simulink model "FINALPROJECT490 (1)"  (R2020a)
settings: Solver=VariableStepAuto  StartTime=0.0  StopTime=4/60  RelTol=1e-3
libraries: powerlib x11, powerlib_meascontrol x9

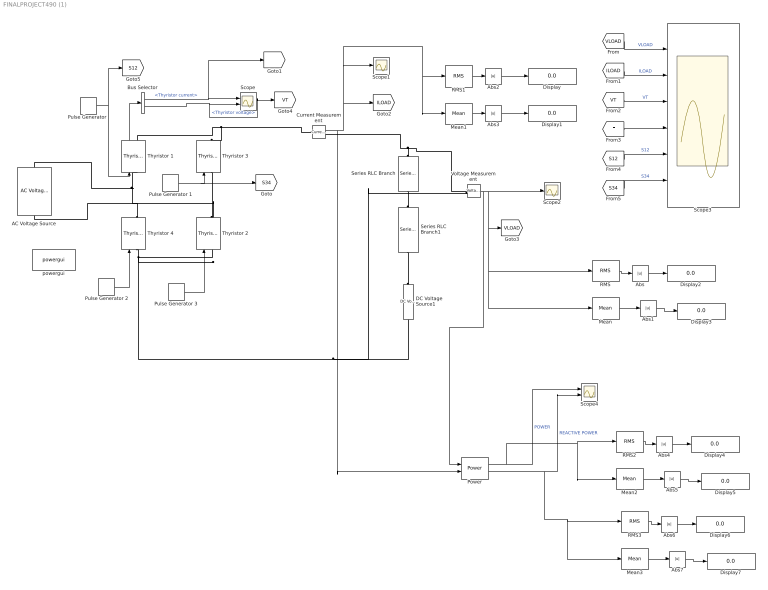
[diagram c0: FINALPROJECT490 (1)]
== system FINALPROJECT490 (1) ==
  "AC Voltage Source " : powerlib/Electrical Sources/AC Voltage Source  Amplitude=169.7  Phase=0  Frequency=60  SampleTime=0  Measurements=None  BusType=swing  Pref=10e3  Qref=0  Qmin=-inf  Qmax=+inf
  Abs{,1..7} (8 alike) : Abs
  Bus Selector : BusSelector  OutputSignals=Thyristor current,Thyristor voltage
  Current Measurement : powerlib/Measurements/Current Measurement  PhasorSimulation=off  OutputType=Complex  PSBequivalent=0
  DC Voltage Source1 : powerlib/Electrical Sources/DC Voltage Source  Amplitude=100  Measurements=None
  Display{,1..7} (8 alike) : Display
  Mean{,1..3} (4 alike) : powerlib_meascontrol/Measurements/Mean  Freq=60  Vinit=0  Ts=0
  Power : powerlib_meascontrol/Measurements/Power  Freq=60  Vinit=[1, 0]  Iinit=[1, 0]  Ts=0
  "Pulse Generator " : DiscretePulseGenerator  PulseType=Time based  Amplitude=5  Period=1/60  PulseWidth=0.51/60  PhaseDelay=((141/360)/60)
  Pulse Generator 1 : DiscretePulseGenerator  PulseType=Time based  Amplitude=5  Period=1/60  PulseWidth=0.51/60  PhaseDelay=(141/360/60)+(0.5/60)
  Pulse Generator 2 : DiscretePulseGenerator  PulseType=Time based  Amplitude=5  Period=1/60  PulseWidth=0.51/60  PhaseDelay=(141/360/60)+(0.5/60)
  Pulse Generator 3 : DiscretePulseGenerator  PulseType=Time based  Amplitude=5  Period=1/60  PulseWidth=0.51/60  PhaseDelay=((141/360)/60)
  RMS{,1..3} (4 alike) : powerlib_meascontrol/Measurements/RMS  TrueRMS=on  Freq=60  RMSInit=120  Ts=0
  Scope : Scope  NumInputPorts=2
  Scope1 : Scope
  Scope2 : Scope
  Scope3 : Scope  NumInputPorts=6
  Scope4 : Scope  NumInputPorts=2
  Series RLC Branch : powerlib/Elements/Series RLC Branch  LConnTagsString=__new0  RConnTagsString=__new0  BranchType=R  Resistance=0.8  Inductance=1e-3  SetiL0=off  InitialCurrent=0  Capacitance=1e-6  Setx0=off  InitialVoltage=0  Measurements=None
  Series RLC Branch1 : powerlib/Elements/Series RLC Branch  LConnTagsString=__new0  RConnTagsString=__new0  BranchType=L  Resistance=20  Inductance=.117  SetiL0=off  InitialCurrent=0  Capacitance=1e-6  Setx0=off  InitialVoltage=0  Measurements=None
  "Thyristor 1 " : powerlib/Power Electronics/Thyristor  Ron=0.001  Lon=0  Vf=0.001  IC=0  Rs=0  Cs=0  Measurements=on
  "Thyristor 2 " : powerlib/Power Electronics/Thyristor  Ron=0.001  Lon=0  Vf=0.001  IC=0  Rs=0  Cs=0  Measurements=on
  "Thyristor 3 " : powerlib/Power Electronics/Thyristor  Ron=0.001  Lon=0  Vf=0.001  IC=0  Rs=0  Cs=0  Measurements=on
  "Thyristor 4 " : powerlib/Power Electronics/Thyristor  Ron=0.001  Lon=0  Vf=0.001  IC=0  Rs=0  Cs=0  Measurements=on
  Voltage Measurement : powerlib/Measurements/Voltage Measurement  PhasorSimulation=off  OutputType=Complex  PSBequivalent=0
  powergui : powerlib/powergui  Priority=1  SimulationMode=Continuous  SampleTime=50e-6  frequency=60  Iterations=50  frequencyindice=60  Pbase=100e6  ErrMax=1e-4  UnitsV=kV  UnitsW=MW  buscounter=0  FunctionMessages=off  echomessages=off  EnableUseOfTLC=off  CurrentSourceSwitches=off  DisableSnubberDevices=off  DisableRonSwitches=off  DisableVfSwitches=off  DisplayEquations=off  AutomaticDiscreteSolvers=off  SolverType=Tustin/Backward Euler (TBE)  Interpol=off  ExternalGateDelay=off  methode=off  Ts=100  x0status=blocks  SPID=on  SwTol=0  HookPort=off  NonlinearTolerance=1e-4  nMaxIteration=100  ContinueOnMaxIteration=off  RestoreLinks=warning  ResistiveCurrentMeasurement=off  Frange=[0:2:500]  Ylog=off  Xlog=on  ShowGrid=off  save=off  variable=ZData  structure=Scope6inputs  ZoomFFT=off  StartTime=0.0  cycles=1  DisplayStyle=4  fundamental=60  FreqAxis=off  MaxFrequency=1000  frequencyindicesteady=1  RmsSteady=1  display=off
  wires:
  Pulse Generator 1/1 -> [S34], "Thyristor 3 "/1
  "Pulse Generator "/1 -> [S12], "Thyristor 1 "/1
  RMS1/1 -> Abs2/1
  Pulse Generator 3/1 -> "Thyristor 2 "/1
  Pulse Generator 2/1 -> "Thyristor 4 "/1
  Abs3/1 -> Display1/1
  Mean1/1 -> Abs3/1
  Bus Selector/1 -> [IT], Scope/1  "<Thyristor current>"
  Abs2/1 -> Display/1
  [ILOAD] -> Scope3/2  "ILOAD"
  RMS/1 -> Abs/1
  [IT] -> Scope3/4  "IT"
  [S34] -> Scope3/6  "S34"
  Bus Selector/2 -> [VT], Scope/2  "<Thyristor voltage>"
  Current Measurement/1 -> Power/2, Scope1/1, Mean1/1, RMS1/1, [ILOAD]
  "Thyristor 1 "/1 -> Bus Selector/1
  [VT] -> Scope3/3  "VT"
  Abs/1 -> Display2/1
  [VLOAD] -> Scope3/1  "VLOAD"
  Voltage Measurement/1 -> Scope2/1, Mean/1, RMS/1, [VLOAD], Power/1
  [S12] -> Scope3/5  "S12"
  Mean/1 -> Abs1/1
  Abs1/1 -> Display3/1
  Abs4/1 -> Display4/1
  RMS2/1 -> Abs4/1
  Abs5/1 -> Display5/1
  Mean2/1 -> Abs5/1
  RMS3/1 -> Abs6/1
  Abs7/1 -> Display7/1
  Abs6/1 -> Display6/1
  Mean3/1 -> Abs7/1
  Power/1 -> Mean2/1, RMS2/1, Scope4/1  "POWER"
  Power/2 -> Mean3/1, RMS3/1, Scope4/2  "REACTIVE POWER"
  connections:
  "Thyristor 4 "/LConn1 -- "Thyristor 2 "/LConn1 -- Voltage Measurement/LConn2 -- DC Voltage Source1/RConn1
  Current Measurement/LConn1 -- "Thyristor 3 "/RConn1 -- "Thyristor 1 "/RConn1
  Series RLC Branch/LConn1 -- Current Measurement/RConn1 -- Voltage Measurement/LConn1
  "Thyristor 2 "/RConn1 -- "Thyristor 3 "/LConn1 -- "AC Voltage Source "/LConn1
  "Thyristor 4 "/RConn1 -- "AC Voltage Source "/RConn1 -- "Thyristor 1 "/LConn1
  Series RLC Branch1/LConn1 -- Series RLC Branch/RConn1
  DC Voltage Source1/LConn1 -- Series RLC Branch1/RConn1
